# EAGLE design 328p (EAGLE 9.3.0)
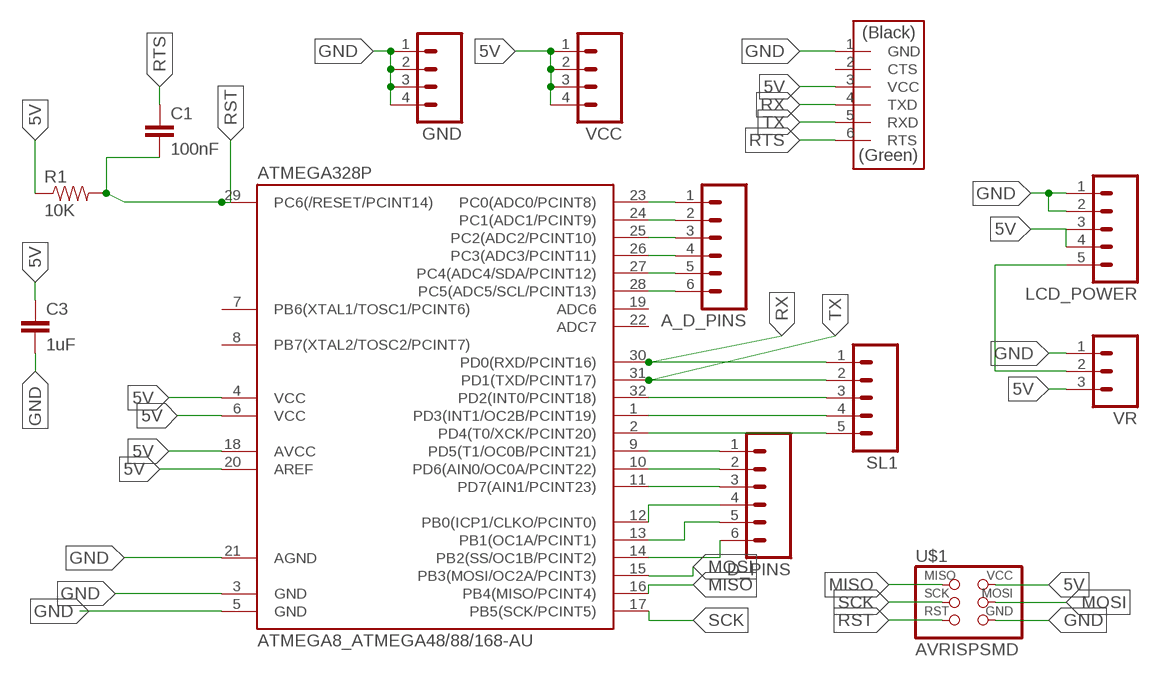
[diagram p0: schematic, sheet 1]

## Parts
A_D_PINS  M06  [06P]
ATMEGA328P  ATMEGA8_ATMEGA48/88/168-AU  [ATMEGA8_TQFP32-08]
C1  100nF  01_SPARKFUN_CAP1206  [01_SPARKFUN_1206]
C3  1uF  01_SPARKFUN_CAP1206  [01_SPARKFUN_1206]
D_PINS  M06  [06P]
GND  M04  [04P]
LCD_POWER  M05  [05P]
R1  10K  01_SPARKFUN_RESISTOR1206  [01_SPARKFUN_1206]
SL1  M05  [05P]
U$1  AVRISPSMD  [2X03SMD]
U$2  FTDI-SMD-HEADER  [1X06SMD]
VCC  M04  [04P]
VR  M03  [03P]

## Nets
5V: ATMEGA328P.4(VCC) ATMEGA328P.6(VCC) ATMEGA328P.18(AVCC) ATMEGA328P.20(AREF) C3.1 LCD_POWER.3 LCD_POWER.4 R1.1 U$1.2(VCC) U$2.3(VCC) VCC.1 VCC.2 VCC.3 VCC.4 VR.3
GND: ATMEGA328P.3(GND) ATMEGA328P.5(GND) ATMEGA328P.21(AGND) C3.2 GND.1 GND.2 GND.3 GND.4 LCD_POWER.1 LCD_POWER.2 U$1.6(GND) U$2.1(GND) VR.1
MISO: ATMEGA328P.16(PB4(MISO/PCINT4)) U$1.1(MISO)
MOSI: ATMEGA328P.15(PB3(MOSI/OC2A/PCINT3)) U$1.4(MOSI)
N$1: ATMEGA328P.9(PD5(T1/OC0B/PCINT21)) D_PINS.1
N$2: ATMEGA328P.10(PD6(AIN0/OC0A/PCINT22)) D_PINS.2
N$3: ATMEGA328P.11(PD7(AIN1/PCINT23)) D_PINS.3
N$4: ATMEGA328P.12(PB0(ICP1/CLKO/PCINT0)) D_PINS.4
N$5: ATMEGA328P.13(PB1(OC1A/PCINT1)) D_PINS.5
N$6: ATMEGA328P.14(PB2(SS/OC1B/PCINT2)) D_PINS.6
N$7: A_D_PINS.1 ATMEGA328P.23(PC0(ADC0/PCINT8))
N$8: A_D_PINS.2 ATMEGA328P.24(PC1(ADC1/PCINT9))
N$9: A_D_PINS.3 ATMEGA328P.25(PC2(ADC2/PCINT10))
N$10: A_D_PINS.4 ATMEGA328P.26(PC3(ADC3/PCINT11))
N$11: A_D_PINS.5 ATMEGA328P.27(PC4(ADC4/SDA/PCINT12))
N$12: A_D_PINS.6 ATMEGA328P.28(PC5(ADC5/SCL/PCINT13))
N$15: ATMEGA328P.32(PD2(INT0/PCINT18)) SL1.3
N$16: ATMEGA328P.1(PD3(INT1/OC2B/PCINT19)) SL1.4
N$17: ATMEGA328P.2(PD4(T0/XCK/PCINT20)) SL1.5
N$20: LCD_POWER.5 VR.2
RST: ATMEGA328P.29(PC6(/RESET/PCINT14)) C1.2 R1.2 U$1.5(RST)
RTS: C1.1 U$2.6(RTS)
RX: ATMEGA328P.30(PD0(RXD/PCINT16)) SL1.1 U$2.4(TXD)
SCK: ATMEGA328P.17(PB5(SCK/PCINT5)) U$1.3(SCK)
TX: ATMEGA328P.31(PD1(TXD/PCINT17)) SL1.2 U$2.5(RXD)
Unconnected: ATMEGA328P.7(PB6(XTAL1/TOSC1/PCINT6)) ATMEGA328P.8(PB7(XTAL2/TOSC2/PCINT7)) ATMEGA328P.19(ADC6) ATMEGA328P.22(ADC7) U$2.2(CTS)

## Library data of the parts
A_D_PINS D_PINS = con-amp-quick:M06: AMP QUICK CONNECTOR; OC_FARNELL: unknown; OC_NEWARK: unknown
ATMEGA328P = satshakit_cnc:ATMEGA8_ATMEGA48/88/168
C1 C3 = satshakit_cnc:01_SPARKFUN_CAP: Capacitor
GND VCC = con-amp-quick:M04: AMP QUICK CONNECTOR; OC_FARNELL: unknown; OC_NEWARK: unknown
LCD_POWER SL1 = con-amp-quick:M05: AMP QUICK CONNECTOR; OC_FARNELL: unknown; OC_NEWARK: unknown
R1 = satshakit_cnc:01_SPARKFUN_RESISTOR: Resistor
U$1 = fab:AVRISP
U$2 = fab:FTDI-SMD-HEADER
VR = con-amp-quick:M03: AMP QUICK CONNECTOR; OC_FARNELL: unknown; OC_NEWARK: unknown

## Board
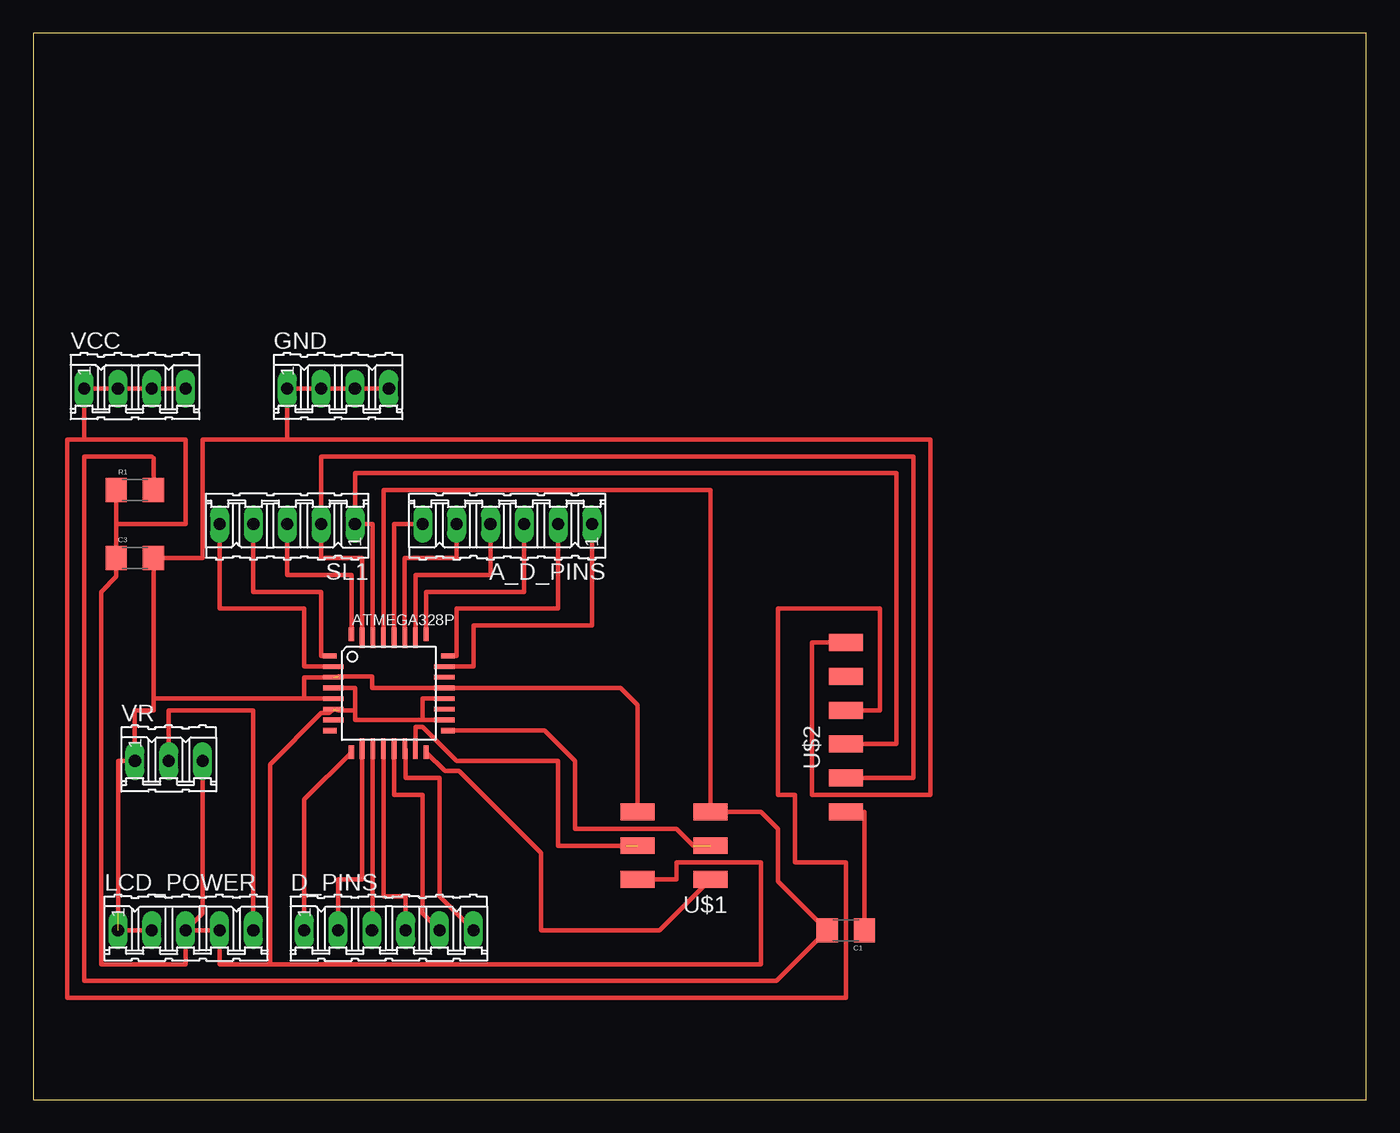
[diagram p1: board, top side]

Size 100 x 80 mm. Coordinates in mm from the lower left corner, seen from the top.
Outline: 0,0 100,0 100,80 0,80 0,0
Copper layers (1*16): Top 0.035mm / dielectric 1.5mm / Bottom 0.035mm
Design rules "default": minimum track width 6mil, minimum drill 0.35mm, track to track 6mil, track to pad 6mil, pad to pad 6mil, via to via 6mil, smd to smd 6mil, copper to edge 40mil, drill to drill 6mil, minimum pad ring 10mil, minimum via ring 8mil, stop-mask expansion 4mil, vias tented up to drill 0mil, thermal gap 10mil

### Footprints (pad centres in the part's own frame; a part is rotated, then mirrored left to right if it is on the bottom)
06P = drill 0.914 long: 1 -6.35,0; 2 -3.81,0; 3 -1.27,0; 4 1.27,0; 5 3.81,0; 6 6.35,0
ATMEGA8_TQFP32-08 = smd 1.016 x 0.406: 1 -4.42,2.8; 8 -4.42,-2.8; 17 4.42,-2.8; 24 4.42,2.8 | smd 1.524 x 0.356: 2 -4.166,2; 3 -4.166,1.2; 4 -4.166,0.4; 5 -4.166,-0.4; 6 -4.166,-1.2; 7 -4.166,-2; 18 4.166,-2; 19 4.166,-1.2; 20 4.166,-0.4; 21 4.166,0.4; 22 4.166,1.2; 23 4.166,2 | smd 0.406 x 1.016: 9 -2.8,-4.42; 16 2.8,-4.42; 25 2.8,4.42; 32 -2.8,4.42 | smd 0.356 x 1.524: 10 -2,-4.166; 11 -1.2,-4.166; 12 -0.4,-4.166; 13 0.4,-4.166; 14 1.2,-4.166; 15 2,-4.166; 26 2,4.166; 27 1.2,4.166; 28 0.4,4.166; 29 -0.4,4.166; 30 -1.2,4.166; 31 -2,4.166
01_SPARKFUN_1206 = smd 1.6 x 1.8: 1 -1.4,0; 2 1.4,0
04P = drill 0.914 long: 1 -3.81,0; 2 -1.27,0; 3 1.27,0; 4 3.81,0
05P = drill 0.914 long: 1 -5.08,0; 2 -2.54,0; 3 0,0; 4 2.54,0; 5 5.08,0
2X03SMD = smd 2.54 x 1.27: 1 -2.54,2.54; 2 2.92,2.54; 3 -2.54,0; 4 2.92,0; 5 -2.54,-2.54; 6 2.92,-2.54
1X06SMD = smd 2.54 x 1.27: 1 0,6.35; 2 0,3.81; 3 0,1.27; 4 0,-1.27; 5 0,-3.81; 6 0,-6.35
03P = drill 0.914 long: 1 -2.54,0; 2 0,0; 3 2.54,0

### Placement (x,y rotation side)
A_D_PINS  35.56,43.18 180 top
ATMEGA328P  26.67,30.48 0 top
C1  60.96,12.7 180 top
C3  7.62,40.64 0 top
D_PINS  26.67,12.7 0 top
GND  22.86,53.34 0 top
LCD_POWER  11.43,12.7 0 top
R1  7.62,45.72 0 top
SL1  19.05,43.18 180 top
U$1  48.26,19.05 180 top
U$2  60.96,27.94 0 top
VCC  7.62,53.34 0 top
VR  10.16,25.4 0 top

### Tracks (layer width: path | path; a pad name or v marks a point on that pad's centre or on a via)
5V  (1 unrouted)
  Top 0.356: ATMEGA328P.4 24.13,30.88 24.13,29.21 | 24.13,29.21 22.86,29.21 | ATMEGA328P.18 29.21,28.48 | 29.21,28.48 24.13,28.48 24.13,29.21 | ATMEGA328P.20 29.21,30.08 29.21,28.48 | 44.45,16.51 U$1.2 48.26,16.51 48.26,17.78 54.61,17.78 54.61,10.16 17.78,10.16 | VR.3 12.7,13.97 LCD_POWER.3 | 6.22,43.18 C3.1 6.22,39.24 5.08,38.1 5.08,10.16 11.43,10.16 LCD_POWER.3 | 6.22,43.18 R1.1 | LCD_POWER.3 LCD_POWER.4 13.97,10.16 17.78,10.16 | ATMEGA328P.6 22.21,28.99 21.61,28.99 17.78,25.16 17.78,10.16 | U$2.3 63.5,29.21 63.5,36.83 55.88,36.83 55.88,22.86 57.15,22.86 57.15,17.78 60.96,17.78 60.96,7.62 2.54,7.62 2.54,49.53 3.81,49.53 | 6.22,43.18 11.43,43.18 11.43,49.53 3.81,49.53 | 3.81,49.53 VCC.1 VCC.2 VCC.3 VCC.4
GND  (2 unrouted)
  Top 0.356: 6.35,13.97 6.35,25.4 VR.1 7.62,29.21 9.02,29.21 9.02,30.08 | 9.02,30.08 C3.2 12.7,40.64 12.7,49.53 19.05,49.53 | ATMEGA328P.5 20.32,30.08 | 20.32,30.08 9.02,30.08 | ATMEGA328P.3 20.32,31.68 20.32,30.08 | 22.86,31.75 25.4,31.75 25.4,30.88 ATMEGA328P.21 44.05,30.88 45.34,29.59 U$1.6 | LCD_POWER.1 LCD_POWER.2 | U$2.1 58.42,34.29 58.42,22.86 67.31,22.86 67.31,49.53 19.05,49.53 | 19.05,49.53 GND.1 GND.2 GND.3 GND.4
MISO
  Top 0.356: U$1.1 46.99,12.7 38.1,12.7 38.1,18.5 31.96,24.64 30.89,24.64 ATMEGA328P.16
MOSI  (1 unrouted)
  Top 0.356: ATMEGA328P.15 28.67,27.94 29.21,27.94 31.75,25.4 39.37,25.4 39.37,19.05 44.45,19.05
N$1
  Top 0.356: D_PINS.1 20.32,22.51 ATMEGA328P.9
N$2
  Top 0.356: ATMEGA328P.10 24.67,16.51 22.86,16.51 D_PINS.2
N$3
  Top 0.356: ATMEGA328P.11 25.47,12.7 D_PINS.3
N$4
  Top 0.356: ATMEGA328P.12 26.27,15.24 27.94,15.24 D_PINS.4
N$5
  Top 0.356: ATMEGA328P.13 27.07,22.86 29.21,22.86 29.21,13.97 D_PINS.5
N$6
  Top 0.356: ATMEGA328P.14 27.94,26.31 27.94,24.13 30.48,24.13 30.48,15.24 D_PINS.6
N$7
  Top 0.356: ATMEGA328P.23 33.02,32.48 33.02,35.56 41.91,35.56 A_D_PINS.1
N$8
  Top 0.356: ATMEGA328P.24 31.75,33.28 31.75,36.83 39.37,36.83 A_D_PINS.2
N$9
  Top 0.356: ATMEGA328P.25 29.47,38.1 36.83,38.1 A_D_PINS.3
N$10
  Top 0.356: ATMEGA328P.26 28.67,39.37 34.29,39.37 A_D_PINS.4
N$11
  Top 0.356: A_D_PINS.5 31.75,40.64 27.87,40.64 ATMEGA328P.27
N$12
  Top 0.356: A_D_PINS.6 27.07,43.18 ATMEGA328P.28
N$15
  Top 0.356: ATMEGA328P.32 23.87,39.37 19.05,39.37 SL1.3
N$16
  Top 0.356: ATMEGA328P.1 21.59,33.28 21.59,38.1 16.51,38.1 SL1.4
N$17
  Top 0.356: ATMEGA328P.2 20.32,32.48 20.32,36.83 13.97,36.83 SL1.5
N$20
  Top 0.356: VR.2 10.16,29.21 16.51,29.21 LCD_POWER.5
RST
  Top 0.356: ATMEGA328P.29 26.27,45.72 50.8,45.72 U$1.5 54.61,21.59 55.88,20.32 55.88,16.38 C1.2 55.75,8.89 3.81,8.89 3.81,48.26 8.89,48.26 9.02,48.13 R1.2
RTS
  Top 0.356: C1.1 62.36,21.59 U$2.6
RX
  Top 0.356: ATMEGA328P.30 25.47,43.18 SL1.1 24.13,46.99 64.77,46.99 64.77,26.67 U$2.4
SCK  (1 unrouted)
  Top 0.356: ATMEGA328P.17 38.36,27.68 40.64,25.4 40.64,20.32 48.26,20.32 49.53,19.05
TX
  Top 0.356: ATMEGA328P.31 24.67,40.64 21.59,40.64 SL1.2 21.59,48.26 66.04,48.26 66.04,24.13 U$2.5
